PROGRAM MAIN
VAR
	stAxis								:	ST_AXIS_DATA;
	fb_Axis_PTP							:	FB_Axis_PTP;
	fbMutliTurnsEncoderCount			:	FB_MutliTurnsEncoderCount:=(eDataTpye:= 0);// (eUDINT,eDINT) 0/1
	fbSetPosition						:	MC_SetPosition;
	bSetHomePos							:	BOOL;
	tonPower_1S							:	TON:=(IN:= TRUE,PT:=T#1S);
	
	User_Pulse_2s						:	FB_Pulse:=(PT_ON:= T#5S,PT_OFF:=T#5S);
	fbWritePersistentData				:	FB_WritePersistentData;
	
END_VAR
VAR PERSISTENT
	bTest								:	BOOL;
END_VAR

	
tonPower_1S();

fb_Axis_PTP(AXIS:= stAxis);
// 上电延时再触发，NC server 准备好才能触发读取 脉冲当量
fbMutliTurnsEncoderCount(
	bExecute:= tonPower_1S.Q AND bTest, // 判断可执行条件：SEW驱动无报错，或使用开机1秒后即可
	refAxis:= stAxis.AXIS_REF, 
	eDataTpye:= , 
	Numerator=> , 
	Denominator=> , 
	SetPosition=> , 
	sLog=> , 
	bBusy=> , 
	bError=> );
// 手动设置位置，包括但不限于原点
fbSetPosition.Options.ClearPositionLag := TRUE;// 清除跟随误差
fbSetPosition(
	Axis:= stAxis.AXIS_REF, 
	Execute:= bSetHomePos, 
	Position:= 0, 
	Mode:= , (* RELATIVE=True, ABSOLUTE=False (Default) *)
	Options:= , 
	Done=> , 
	Busy=> , 
	Error=> , 
	ErrorID=> );
// 初始化完成标记位
IF tonPower_1S.Q 
AND NOT fbMutliTurnsEncoderCount.bBusy 
AND NOT fbMutliTurnsEncoderCount.bError THEN 
	;
END_IF

User_Pulse_2s(IN:= tonPower_1S.Q);
fbWritePersistentData(
	NETID:= , 
	PORT:= 851, 
	START:= User_Pulse_2s.Q, 
	TMOUT:= , 
	MODE:= , 
	BUSY=> , 
	ERR=> , 
	ERRID=> );

END_PROGRAM
